| TEXAS INSTRUMENTS INCORPORATED
| Standard Linear and Logic Group
| IBIS Model of SN74AHC08
| QUADRUPLE 2-INPUT POSITIVE-AND GATES
| This file contains package information for the following:
|  SOIC 14-pin (D) package as [Component] AHC08_D
|  SSOP 14-pin (DB) package as [Component] AHC08_DB
|  TVSOP 14-pin (DGV) package as [Component] AHC08_DGV
|  PDIP 14-pin (N) package as [Component] AHC08_N
|  SOP 14-pin (NS) package as [Component] AHC08_NS
|  TSSOP 14-pin (PW) package as [Component] AHC08_PW
| This device can be powered at the following Vccs:
|  2.2 volt Vcc
|  3.3 volt Vcc
|  5 volt Vcc
| This file provides unique models under the [Model Selector] for each Vcc.
| For operation at a specific Vcc, select the appropriate model after each
| [Model Selector] keyword.
[IBIS Ver]   3.2
[Comment char]  |_char
[File Name]   sn74ahc08.ibs
[File Rev]   1.1  b_die
[Date]   May 13, 2002
[Source]   Data created from TI-SPICE simulations at TI-SLL.
[Notes]   The following is an IBIS list for the AHC08.
   Please contact sllibis@ti.com with questions and
   comments concerning SLL IBIS models.
   -C_comp values are taken at a different test condition
   than the data sheet.
[Disclaimer] Property of Texas Instruments Incorporated.  Unauthorized
   reproduction and/or distribution is strictly prohibited.
   This product is protected under copyright law.
   Created  2002, (C) Copyright  2002, Texas Instruments
   Incorporated, All Rights Reserved
   UNLESS THERE IS A SIGNED, WRITTEN AGREEMENT TO THE
   CONTRARY, TEXAS INSTRUMENTS (TI) IS PROVIDING THE IBIS
   MODELS  AND WITHOUT ANY WARRANTY, EXPRESSED OR
   IMPLIED.  TI assumes no liability for:
   1) the accuracy of the IBIS models provided to your
   company;
   2) the proper functioning of these IBIS Models in your
   design or for any resulting applications; or
   3) infringement of patents, copyrights or intellectual
   property rights resulting from your use of these IBIS
   models.
   TI provides IBIS Models as a service to our customers.
   You and your company shall not distribute, sell or give
   these models to anyone else without prior written
   permission from TI.
   TI reserves the right to make changes to our products or
   to discontinue any semiconductor product or service
   without notice, and advises our customers to obtain the
   latest version of relevant information to verify, before
   placing orders, that the information being relied on is
   current.
   Please be aware that your receipt and use of the IBIS
   information provided shall serve as acceptance of these
   terms and conditions.  If you do not accept these terms,
   you should return or destroy the IBIS models and any
   other accompanying information immediately.
| Component AHC08_D 14-pin SOIC
[Component]   AHC08_D
[Manufacturer]   Texas Instruments, Inc.
[Package]
|   typ   min   max
R_pkg   3.100e-02   2.800e-02   3.400e-02
L_pkg   3.109e-09   2.462e-09   3.889e-09
C_pkg   4.730e-13   3.630e-13   6.280e-13
[Pin]   signal_name   model_name   R_pin   L_pin   C_pin
1   1A   AHC08_IN   3.300e-02   3.854e-09   6.220e-13
2   1B   AHC08_IN   3.200e-02   3.188e-09   4.730e-13
3   1Y   AHC08_OUT   2.800e-02   2.462e-09   3.770e-13
4   2A   AHC08_IN   3.100e-02   2.596e-09   3.630e-13
5   2B   AHC08_IN   2.800e-02   2.521e-09   3.720e-13
6   2Y   AHC08_OUT   3.400e-02   3.250e-09   4.760e-13
7   GND   GND   3.400e-02   3.889e-09   6.280e-13
8   3Y   AHC08_OUT   3.400e-02   3.889e-09   6.280e-13
9   3A   AHC08_IN   3.400e-02   3.250e-09   4.760e-13
10   3B   AHC08_IN   2.800e-02   2.521e-09   3.720e-13
11   4Y   AHC08_OUT   3.100e-02   2.596e-09   3.640e-13
12   4A   AHC08_IN   2.800e-02   2.462e-09   3.770e-13
13   4B   AHC08_IN   3.200e-02   3.188e-09   4.730e-13
14   VCC   POWER   3.300e-02   3.854e-09   6.220e-13
| Component AHC08_DB 14-pin SSOP
[Component]   AHC08_DB
[Manufacturer]   Texas Instruments, Inc.
[Package]
|   typ   min   max
R_pkg   4.400e-02   4.100e-02   4.600e-02
L_pkg   3.551e-09   3.258e-09   3.927e-09
C_pkg   4.020e-13   3.600e-13   4.210e-13
[Pin]   signal_name   model_name   R_pin   L_pin   C_pin
1   1A   AHC08_IN   4.600e-02   3.927e-09   4.080e-13
2   1B   AHC08_IN   4.400e-02   3.587e-09   4.210e-13
3   1Y   AHC08_OUT   4.100e-02   3.289e-09   3.980e-13
4   2A   AHC08_IN   4.200e-02   3.258e-09   3.600e-13
5   2B   AHC08_IN   4.100e-02   3.286e-09   4.030e-13
6   2Y   AHC08_OUT   4.400e-02   3.586e-09   4.210e-13
7   GND   GND   4.600e-02   3.927e-09   4.080e-13
8   3Y   AHC08_OUT   4.600e-02   3.927e-09   4.080e-13
9   3A   AHC08_IN   4.400e-02   3.586e-09   4.210e-13
10   3B   AHC08_IN   4.100e-02   3.286e-09   4.030e-13
11   4Y   AHC08_OUT   4.300e-02   3.258e-09   3.600e-13
12   4A   AHC08_IN   4.100e-02   3.289e-09   3.980e-13
13   4B   AHC08_IN   4.400e-02   3.587e-09   4.210e-13
14   VCC   POWER   4.600e-02   3.927e-09   4.080e-13
| Component AHC08_DGV 14-pin TVSOP
[Component]   AHC08_DGV
[Manufacturer]   Texas Instruments, Inc.
[Package]
|   typ   min   max
R_pkg   3.500e-02   2.000e-02   4.500e-02
L_pkg   2.499e-09   2.077e-09   2.966e-09
C_pkg   3.610e-13   3.050e-13   4.160e-13
[Pin]   signal_name   model_name   R_pin   L_pin   C_pin
1   1A   AHC08_IN   2.700e-02   2.717e-09   3.730e-13
2   1B   AHC08_IN   3.700e-02   2.434e-09   3.980e-13
3   1Y   AHC08_OUT   3.400e-02   2.200e-09   3.160e-13
4   2A   AHC08_IN   2.000e-02   2.077e-09   3.090e-13
5   2B   AHC08_IN   3.000e-02   2.147e-09   3.050e-13
6   2Y   AHC08_OUT   4.200e-02   2.580e-09   4.080e-13
7   GND   GND   3.900e-02   2.921e-09   3.850e-13
8   3Y   AHC08_OUT   3.300e-02   2.841e-09   3.800e-13
9   3A   AHC08_IN   4.200e-02   2.611e-09   4.100e-13
10   3B   AHC08_IN   3.800e-02   2.331e-09   3.290e-13
11   4Y   AHC08_OUT   2.600e-02   2.223e-09   3.190e-13
12   4A   AHC08_IN   3.400e-02   2.259e-09   3.130e-13
13   4B   AHC08_IN   4.500e-02   2.681e-09   4.160e-13
14   VCC   POWER   4.200e-02   2.966e-09   3.860e-13
| Component AHC08_N 14-pin PDIP
[Component]   AHC08_N
[Manufacturer]   Texas Instruments, Inc.
[Package]
|   typ   min   max
R_pkg   4.500e-02   3.700e-02   6.300e-02
L_pkg   5.407e-09   3.922e-09   6.942e-09
C_pkg   3.890e-13   2.050e-13   6.040e-13
[Pin]   signal_name   model_name   R_pin   L_pin   C_pin
1   1A   AHC08_IN   6.300e-02   6.942e-09   6.040e-13
2   1B   AHC08_IN   3.700e-02   6.200e-09   4.060e-13
3   1Y   AHC08_OUT   4.200e-02   4.389e-09   3.220e-13
4   2A   AHC08_IN   3.800e-02   3.922e-09   2.050e-13
5   2B   AHC08_IN   3.900e-02   4.301e-09   2.980e-13
6   2Y   AHC08_OUT   3.800e-02   5.329e-09   3.560e-13
7   GND   GND   5.300e-02   6.510e-09   5.440e-13
8   3Y   AHC08_OUT   5.300e-02   6.437e-09   5.390e-13
9   3A   AHC08_IN   3.900e-02   5.352e-09   3.470e-13
10   3B   AHC08_IN   4.200e-02   4.473e-09   2.970e-13
11   4Y   AHC08_OUT   4.400e-02   4.326e-09   2.250e-13
12   4A   AHC08_IN   4.200e-02   4.295e-09   2.800e-13
13   4B   AHC08_IN   4.200e-02   6.318e-09   4.180e-13
14   VCC   POWER   6.100e-02   6.900e-09   6.030e-13
| Component AHC08_NS 14-pin SOP
[Component]   AHC08_NS
[Manufacturer]   Texas Instruments, Inc.
[Package]
|   typ   min   max
R_pkg   4.500e-02   3.900e-02   5.400e-02
L_pkg   3.796e-09   2.561e-09   4.952e-09
C_pkg   5.280e-13   2.880e-13   7.100e-13
[Pin]   signal_name   model_name   R_pin   L_pin   C_pin
1   1A   AHC08_IN   4.700e-02   4.867e-09   7.060e-13
2   1B   AHC08_IN   5.100e-02   4.083e-09   5.920e-13
3   1Y   AHC08_OUT   4.100e-02   2.915e-09   3.760e-13
4   2A   AHC08_IN   3.900e-02   2.561e-09   2.880e-13
5   2B   AHC08_IN   4.100e-02   3.101e-09   4.300e-13
6   2Y   AHC08_OUT   4.700e-02   4.047e-09   5.890e-13
7   GND   GND   5.100e-02   4.909e-09   7.000e-13
8   3Y   AHC08_OUT   4.500e-02   4.784e-09   6.940e-13
9   3A   AHC08_IN   5.400e-02   4.176e-09   5.970e-13
10   3B   AHC08_IN   3.900e-02   3.287e-09   4.490e-13
11   4Y   AHC08_OUT   3.900e-02   2.586e-09   2.940e-13
12   4A   AHC08_IN   4.000e-02   2.802e-09   3.710e-13
13   4B   AHC08_IN   4.900e-02   4.080e-09   5.930e-13
14   VCC   POWER   5.200e-02   4.952e-09   7.100e-13
| Component AHC08_PW 14-pin TSSOP
[Component]   AHC08_PW
[Manufacturer]   Texas Instruments, Inc.
[Package]
|   typ   min   max
R_pkg   3.200e-02   2.900e-02   3.500e-02
L_pkg   2.378e-09   2.170e-09   2.680e-09
C_pkg   3.140e-13   2.700e-13   3.350e-13
[Pin]   signal_name   model_name   R_pin   L_pin   C_pin
1   1A   AHC08_IN   3.300e-02   2.618e-09   3.300e-13
2   1B   AHC08_IN   3.100e-02   2.313e-09   3.170e-13
3   1Y   AHC08_OUT   3.000e-02   2.310e-09   3.140e-13
4   2A   AHC08_IN   3.100e-02   2.173e-09   2.720e-13
5   2B   AHC08_IN   3.000e-02   2.204e-09   3.090e-13
6   2Y   AHC08_OUT   3.200e-02   2.315e-09   3.170e-13
7   GND   GND   3.500e-02   2.680e-09   3.350e-13
8   3Y   AHC08_OUT   3.300e-02   2.640e-09   3.330e-13
9   3A   AHC08_IN   3.400e-02   2.347e-09   3.190e-13
10   3B   AHC08_IN   2.900e-02   2.277e-09   3.130e-13
11   4Y   AHC08_OUT   3.100e-02   2.170e-09   2.700e-13
12   4A   AHC08_IN   3.100e-02   2.244e-09   3.110e-13
13   4B   AHC08_IN   3.300e-02   2.343e-09   3.210e-13
14   VCC   POWER   3.500e-02   2.657e-09   3.320e-13
| Model AHC08_IN
[Model Selector]   AHC08_IN
AHC08_IN_22   2.2 volt Vcc
AHC08_IN_33   3.3 volt Vcc
AHC08_IN_50   5 volt Vcc
| Model AHC08_OUT
[Model Selector]   AHC08_OUT
AHC08_OUT_22   2.2 volt Vcc
AHC08_OUT_33   3.3 volt Vcc
AHC08_OUT_50   5 volt Vcc
| Models and submodels in the file (6): AHC08_IN_22 (Input), AHC08_IN_33 (Input), AHC08_IN_50 (Input), AHC08_OUT_22 (Output), AHC08_OUT_33 (Output), AHC08_OUT_50 (Output)
